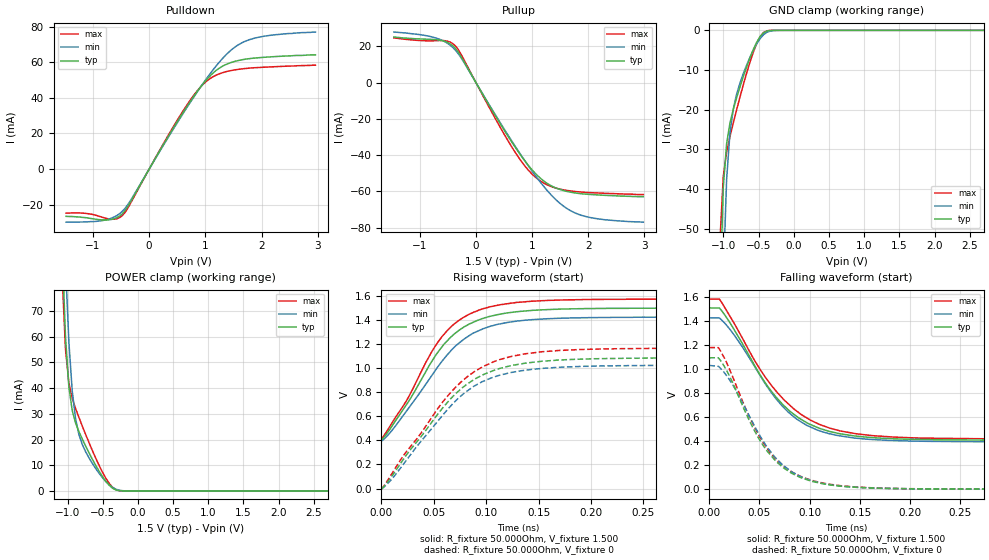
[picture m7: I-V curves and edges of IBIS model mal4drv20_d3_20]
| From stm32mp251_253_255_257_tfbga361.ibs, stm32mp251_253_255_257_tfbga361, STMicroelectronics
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[Model] mal4drv20_d3_20
Model_type   I/O
Polarity   Non-Inverting
Enable   Active-High
C_comp   1.836pF   1.830pF   1.844pF
C_comp_pullup   929.639fF   923.197fF   937.397fF
C_comp_pulldown 781.611fF   776.676fF   790.636fF
Vinh = 885.000mV
Vinl = 615.000mV
Vmeas = 750.000mV
Vref = 750.000mV
Rref = 50Ohms
Cref = 0pF
[Model Spec]
Vinh   885.000mV   848.000mV   923.000mV
Vinl   615.000mV   578.000mV   653.000mV
Vmeas   750.000mV   713.000mV   788.000mV
Vref   750.000mV   713.000mV   788.000mV
D_overshoot_ampl_h 0.4 NA   NA
D_overshoot_ampl_l 0.4 NA   NA
D_overshoot_area_l 100.000m NA   NA
D_overshoot_area_h 100.000m NA   NA
[Receiver Thresholds]
Vth = 750.000mV
Vth_min = 713.000mV
Vth_max = 788.000mV
Vinh_ac = 135.000mV
Vinh_dc = 100.000mV
Vinl_ac = -135.000mV
Vinl_dc = -100.000mV
Tslew_ac = 5.000ns
Threshold_sensitivity = 0.5
Reference_supply Pullup_ref
[Temperature Range]   25.000   125.000   -40.000
[Voltage Range]   1.500V   1.425V   1.575V
[GND Clamp Reference]   0.00V   0.00V   0.00V
[C Comp Corner]
| variable   typ   min   max
C_comp 1.844pF   1.836pF   1.830pF
C_comp_pullup 929.639fF   937.397fF   923.197fF
C_comp_pulldown 776.676fF   790.636fF   781.611fF
[Pulldown Reference]   0.00V   0.00V   0.00V
[POWER Clamp Reference]   1.500V   1.425V   1.575V
[Pullup Reference]   1.500V   1.425V   1.575V
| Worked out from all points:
|   slope of the pulldown table from 0 to 0.225 V, typ, clamps not added: 18.4 ohm
|   slope of the pullup table from 0 to 0.225 V, typ, clamps not added: 18.8 ohm
|   GND clamp passes 1 mA (typ) near -0.45 V on its own axis
|   POWER clamp passes 1 mA (typ) near -0.36 V on its own axis
|   rising waveform, R_fixture 50.000Ohm, V_fixture 1.500: 20-80 % time 51ps typ, 55.1ps min, 48.6ps max; typ from 0.404 V to 1.5 V
|   rising waveform, R_fixture 50.000Ohm, V_fixture 0: 20-80 % time 63.3ps typ, 62.3ps min, 64.9ps max; typ from -0.005 V to 1.09 V
|   falling waveform, R_fixture 50.000Ohm, V_fixture 1.500: 20-80 % time 56ps typ, 54.6ps min, 60.2ps max; typ from 1.51 V to 0.408 V
|   falling waveform, R_fixture 50.000Ohm, V_fixture 0: 20-80 % time 44.5ps typ, 46.2ps min, 45.2ps max; typ from 1.09 V to 0 V
[GND Clamp]
-1.48V    -1.637A    -1.644A    -1.658A
-1.05V    -67.86mA   -111.2mA   -53.06mA
-1.002V   -39.45mA   -62.21mA   -36.77mA
-954.6mV  -28.48mA   -37.5mA    -30.67mA
-906.8mV  -23.32mA   -25.75mA   -26.73mA
-859.1mV  -19.86mA   -19.72mA   -23.25mA
-763.6mV  -14.17mA   -13.2mA    -16.7mA
-668.2mV  -9.09mA    -8.668mA   -10.65mA
-525mV    -2.932mA   -3.341mA   -3.236mA
-429.5mV  -625.7uA   -1.091mA   -535.7uA
-238.6mV  -2.309uA   -20.7uA    -473nA
2.959V    72.19nA    968.6nA    105nA
[Power Clamp]
-1.459V   654.6mA    675.2mA    655.4mA
-1.077V   94.79mA    129.9mA    83.6mA
-1.03V    59.92mA    88.13mA    55.16mA
-981.8mV  40.46mA    57.96mA    42.01mA
-934.1mV  31.26mA    38.88mA    36.03mA
-886.4mV  26.43mA    28.01mA    32.07mA
-838.6mV  23.06mA    21.89mA    28.58mA
-647.7mV  12.32mA    10.7mA     15.7mA
-504.6mV  5.603mA    5.163mA    7.311mA
-361.4mV  1.062mA    1.366mA    1.412mA
-218.2mV  16.86uA    87.94uA    13.19uA
2.98V     -71.2nA    -1.524uA   -71.42nA
[Pulldown]
-1.48V    -26.5mA    -29.8mA    -24.7mA
-1.05V    -27.65mA   -29.5mA    -25.19mA
-763.6mV  -28.57mA   -28.44mA   -27.67mA
-477.3mV  -25.06mA   -23.67mA   -26.11mA
-334.1mV  -18.51mA   -17.76mA   -19.31mA
286.4mV   15.49mA    15.07mA    16.07mA
668.2mV   34.92mA    34.38mA    35.79mA
906.8mV   45.71mA    45.69mA    45.85mA
1.145V    54.16mA    56.04mA    51.99mA
1.48V     60.05mA    67.35mA    55.45mA
1.766V    61.93mA    72.43mA    56.63mA
2.959V    64.1mA     76.9mA     58.3mA
[Pullup]
-1.459V   25.1mA     27.79mA    24.56mA
-743.2mV  23.68mA    24.82mA    23.01mA
-504.6mV  22.07mA    21.59mA    22.77mA
-361.4mV  18.68mA    17.72mA    20.06mA
-265.9mV  14.39mA    13.74mA    15.66mA
688.6mV   -35.18mA   -34.62mA   -37.95mA
927.3mV   -45.45mA   -45.64mA   -48.06mA
1.166V    -53.23mA   -55.66mA   -54.64mA
1.5V      -58.99mA   -66.67mA   -58.75mA
1.834V    -61.13mA   -72.7mA    -60.25mA
2.311V    -62.18mA   -75.66mA   -61.05mA
2.98V     -62.9mA    -76.96mA   -61.74mA
[Ramp]
R_load=50.000Ohm
dV/dt_r   653.670mV/58.500ps  616.799mV/59.500ps  697.140mV/58.000ps
dV/dt_f   653.670mV/50.500ps  616.799mV/51.000ps  697.140mV/53.500ps
[Rising waveform]
R_fixture=50.000Ohm
V_fixture=1.500
V_fixture_min=1.425
V_fixture_max=1.575
0s        403.7mV    393.6mV    412.4mV
9ps       505mV      471.6mV    530.4mV
23ps      685.2mV    633.7mV    716.6mV
48ps      1.056V     939.7mV    1.137V
58ps      1.18V      1.06V      1.265V
78ps      1.339V     1.238V     1.421V
100ps     1.422V     1.337V     1.502V
130ps     1.47V      1.393V     1.548V
175ps     1.492V     1.417V     1.568V
469ps     1.5V       1.425V     1.575V
[Rising waveform]
R_fixture=50.000Ohm
V_fixture=0
0s        -5.252mV   -3.534mV   -4.583mV
8ps       78.98mV    60.02mV    96.04mV
21ps      244.4mV    202.4mV    273.8mV
66ps      745.9mV    685.1mV    797.6mV
77ps      836mV      778.1mV    892.9mV
88ps      903.1mV    849mV      967.4mV
114ps     1.001V     944.2mV    1.075V
149ps     1.054V     995.4mV    1.133V
190ps     1.076V     1.015V     1.156V
469ps     1.086V     1.025V     1.167V
[Falling waveform]
R_fixture=50.000Ohm
V_fixture=1.500
V_fixture_min=1.425
V_fixture_max=1.575
0s        1.509V     1.426V     1.583V
10ps      1.509V     1.426V     1.583V
27ps      1.298V     1.258V     1.348V
48ps      988.2mV    982.6mV    1.032V
72ps      715.4mV    698.6mV    766.3mV
96ps      559.6mV    537.4mV    599.4mV
119ps     482.9mV    463.1mV    511.1mV
145ps     443mV      425.5mV    462.8mV
194ps     416.9mV    402.2mV    429.8mV
479ps     407.5mV    393.9mV    417.8mV
[Falling waveform]
R_fixture=50.000Ohm
V_fixture=0
0s        1.094V     1.03V      1.179V
11ps      1.073V     1.007V     1.153V
24ps      872mV      859.7mV    920.6mV
43ps      518.9mV    557.9mV    548.7mV
61ps      285mV      314.4mV    301.5mV
83ps      128.9mV    140.2mV    140.5mV
100ps     71.15mV    75.64mV    78.77mV
134ps     22.78mV    23.12mV    26.62mV
185ps     4.798mV    4.773mV    5.734mV
478ps     2.785uV    9.279uV    2.243uV
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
